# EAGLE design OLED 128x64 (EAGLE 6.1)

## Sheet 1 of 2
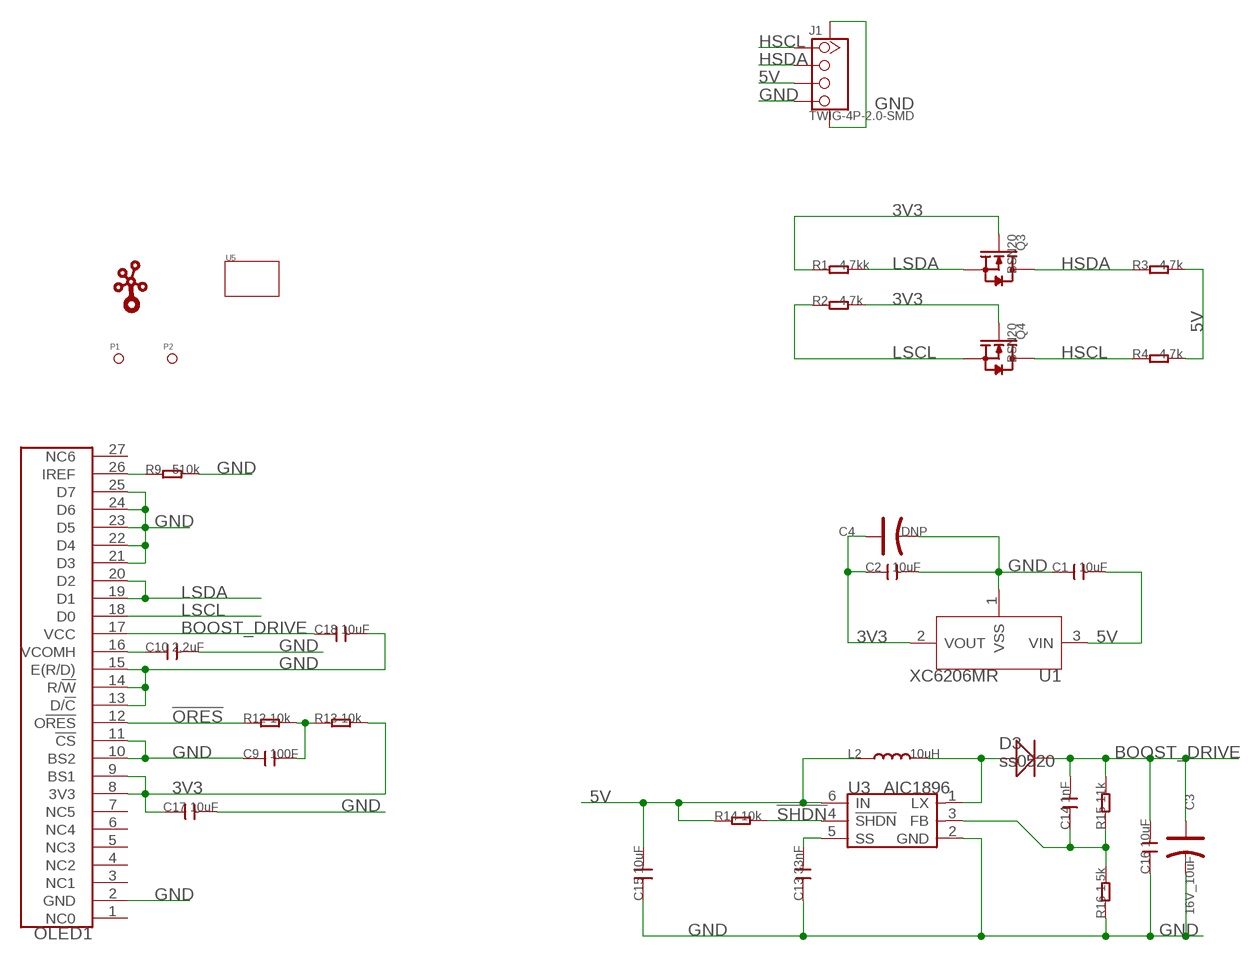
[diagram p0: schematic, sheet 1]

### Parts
C1  10uF  C-0805  [C0805]
C2  10uF  C-0805  [C0805]
C3  16V_10uF  CAP-AVX-A  [AVX-A]
C4  DNP  CAP-AVX-A  [AVX-A]
C9  100F  C-0603  [C0603]
C10  2.2uF  C-0805  [C0805]
C13  33nF  C-0603  [C0603]
C14  1nF  C-0603  [C0603]
C15  10uF  006-C0805  [0805]
C16  10uF  C-0805  [C0805]
C17  10uF  C-0805  [C0805]
C18  10uF  C-0805  [C0805]
D3  ss0520  010-DSOD123  [SOD123]
J1  TWIG-4P-2.0-SMD  TWIG-4P-2.0-SMD-FEMALE-REINFORCE'90D'  [4P-SMD-2.0-90D]
L2  10uH  L'1813'  [1813]
OLED1  OLED_12864BEND  [0LED128X64_BEND]
P1  PAD-MARK  [ROUND-MARK-1.0]
P2  PAD-MARK  [ROUND-MARK-1.0]
Q3  BSN20  MOSFET-N'SOT23'  [SOT23]
Q4  BSN20  MOSFET-N'SOT23'  [SOT23]
R1  4.7kk  R-0603  [R0603]
R2  4.7k  R-0603  [R0603]
R3  4.7k  R-0603  [R0603]
R4  4.7k  R-0603  [R0603]
R9  510k  R-0603  [R0603]
R12  10k  R-0603  [R0603]
R13  10k  R-0603  [R0603]
R14  10k  R-0603  [R0603]
R15  11k  R-0603  [R0603]
R16  1.5k  R-0603  [R0603]
U1  XC6206MR  [SOT23]
U3  AIC1896  [SOT23-6]
U5  TWIG'2U'  [2U-DIM-W/DRILL]
U$1  TWIGLOGOTWIGLOGO_SMALL  [TWIGLOGO_SMALL]

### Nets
3V3: C2.1 C4.+ C17.1 OLED1.8(3V3) OLED1.9(BS1) Q3.1(G) Q4.1(G) R1.1 R2.2 R13.2 U1.2(VOUT)
5V: C1.2 C15.2 J1.3 L2.1 R3.2 R4.2 R14.1 U1.3(VIN) U3.6(IN)
!ORES: OLED1.12(O!RES) R12.1
!SHDN: R14.2 U3.4(!SHDN)
BOOST_DRIVE: C3.+ C14.2 C16.2 C18.1 D3.- OLED1.17(VCC) R15.2
GND: C1.1 C2.2 C3.- C4.- C9.1 C10.2 C13.1 C15.1 C16.1 C17.2 C18.2 J1.4 J1.SS1 J1.SS2 OLED1.2(GND) OLED1.10(BS2) OLED1.11(!CS) OLED1.13(D/!C) OLED1.14(R/!W) OLED1.15(E(R/D)) OLED1.21(D3) OLED1.22(D4) OLED1.23(D5) OLED1.24(D6) OLED1.25(D7) R9.2 R16.1 U1.1(VSS) U3.2(GND)
HSCL: J1.1 Q4.3(D) R4.1
HSDA: J1.2 Q3.3(D) R3.1
LSCL: OLED1.18(D0) Q4.2(S) R2.1
LSDA: OLED1.19(D1) OLED1.20(D2) Q3.2(S) R1.2
N$7: C13.2 U3.5(SS)
N$8: D3.+ L2.2 U3.1(LX)
N$9: C14.1 R15.1 R16.2 U3.3(FB)
N$10: OLED1.26(IREF) R9.1
N$11: C10.1 OLED1.16(VCOMH)
N$12: C9.2 R12.2 R13.1
Unconnected: OLED1.1(NC0) OLED1.3(NC1) OLED1.4(NC2) OLED1.5(NC3) OLED1.6(NC4) OLED1.7(NC5) OLED1.27(NC6)

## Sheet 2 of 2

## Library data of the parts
C1 C2 C9 C10 C13 C14 C16-C18 = Discrete:C*: Ceramic Capacitors
C3 C4 = Discrete:CAP*: Electrolytic Capacitors,Tantalum Capacitors and Super Capacitors
C15 = Discrete:006-C*: Ceramic Capacitors
D3 = Discrete:010-D*
J1 = Connector:TWIG-4P-2.0-SMD-FEMALE-REINFORCE
L2 = Discrete:L*
OLED1 = EXT_moudle:OLED_12864
P1 P2 = Discrete:PAD-MARK; PARTNO: DNP
Q3 Q4 = Discrete:MOSFET-N: IRLL014: http://www.vishay.com/docs/91319/sihll014.pdf
R1-R4 R9 R12-R16 = Discrete:R*
U1 = IC:XC6206: LOW ESR Cap.Compatible Positive Voltage Regulators
U3 = ICs_v54:AIC1896
U5 = moudle:TWIG
U$1 = seeedleo:TWIGLOGO

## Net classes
0 default: width 0.203 mm, drill 0.305 mm, clearance 0.203 mm
1 power: width 0.203 mm, drill 0.305 mm, clearance 0.203 mm
2 gnd: width 0.203 mm, drill 0.305 mm, clearance 0.203 mm
3 usbvcc: width 0.203 mm, drill 0.305 mm, clearance 0.203 mm

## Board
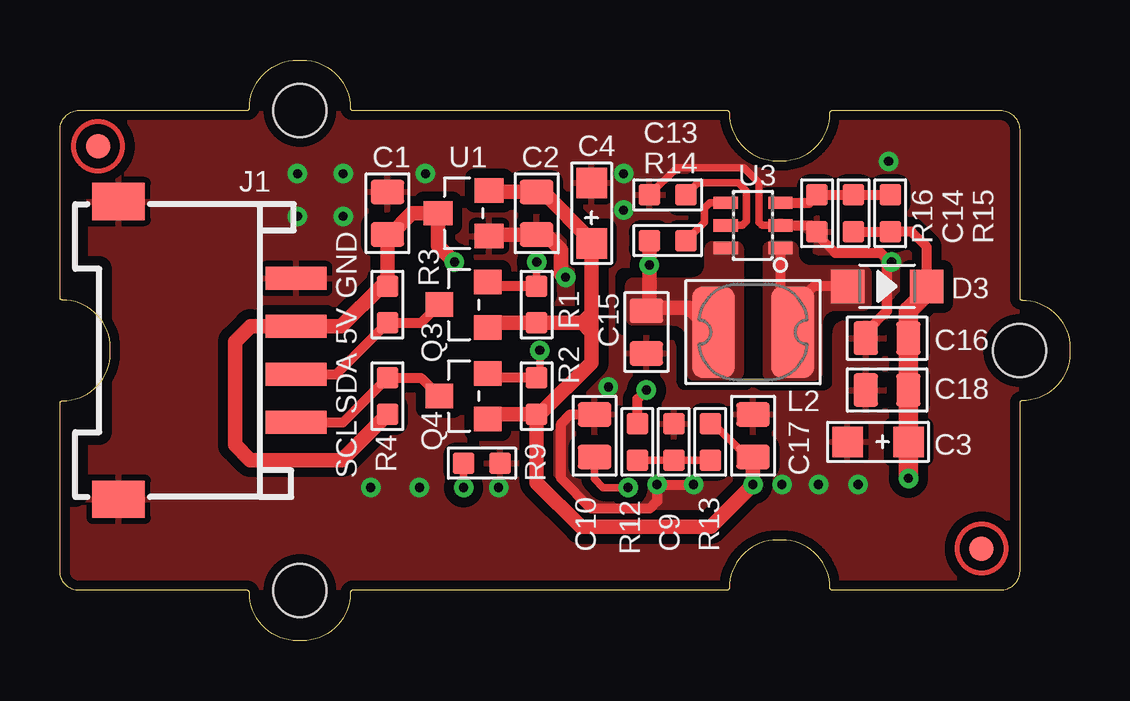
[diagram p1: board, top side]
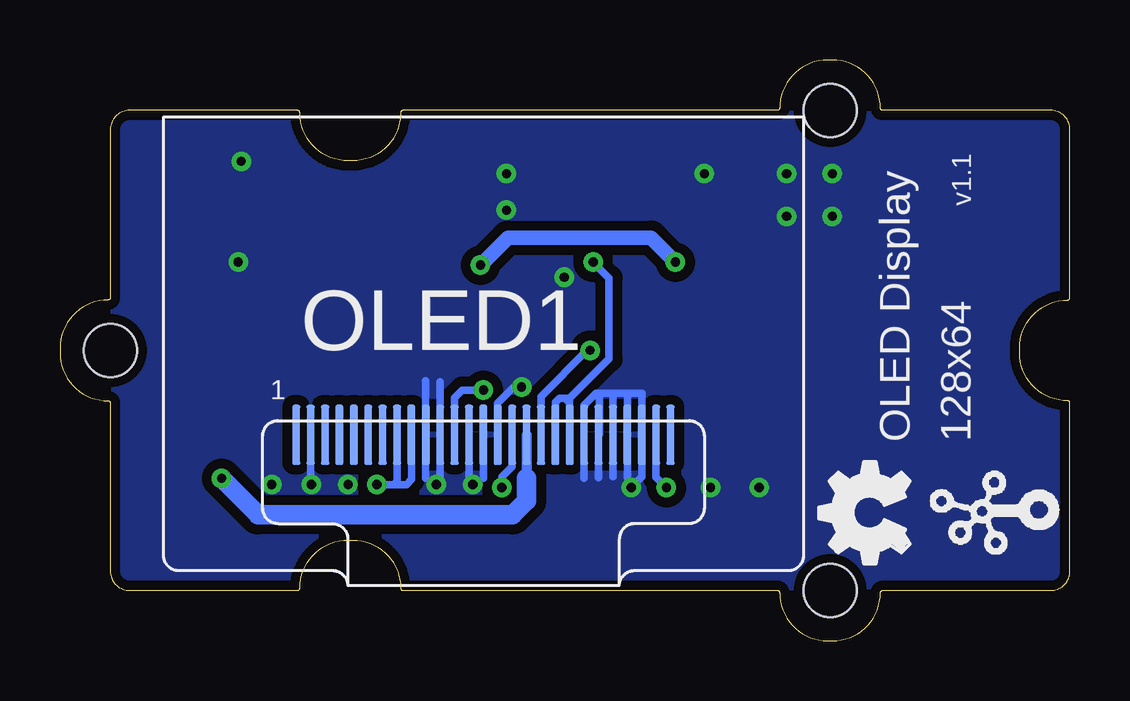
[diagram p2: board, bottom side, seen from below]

Size 42.1 x 24.2 mm. Coordinates in mm from the lower left corner, seen from the top.
Copper layers (1*16): Top 0.035mm / dielectric 1.5mm / Bottom 0.035mm
Design rules: minimum track width 6mil, minimum drill 12mil, track to track 6mil, track to pad 6mil, pad to pad 6mil, via to via 6mil, smd to smd 0mil, copper to edge 10mil, drill to drill 10mil, minimum pad ring 10mil, minimum via ring 6mil, stop-mask expansion 2mil, vias tented up to drill 100mil, thermal gap 10mil
bRestrict: area 24.7,7.9 to 24.8,8.3; area 27.1,7.9 to 27.2,8.3; area 25.3,7.9 to 25.5,8.3; area 18.7,7.9 to 18.9,8.3; area 20.5,7.9 to 20.6,8.3; area 19.9,7.9 to 20,8.3; area 19.4,7.9 to 19.5,8.3; area 38.5,-10.9 to 38.9,-10.6; area 29.5,-15 to 29.9,-14.4; area 27.1,-15 to 28.1,-14.4; area 21,-15 to 23.3,-14.4; area 16.3,-11 to 16.7,-10.5

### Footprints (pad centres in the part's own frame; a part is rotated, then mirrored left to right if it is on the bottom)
C0805 = smd 1.016 x 1.397: 1 -0.889,0; 2 0.889,0
AVX-A = smd 1.27 x 1.27: + -1.27,0; - 1.27,0
C0603 = smd 0.889 x 0.889: 1 -0.762,0; 2 0.762,0
0805 = smd 1.016 x 1.397: 1 -0.889,0; 2 0.889,0
SOD123 = smd 1.397 x 1.397: + 1.651,0; - -1.651,0
4P-SMD-2.0-90D = smd 0.965 x 2.54: 1 -3,0; 2 -1,0; 3 1,0; 4 3,0 | smd 1.55 x 2.184: SS1 -6.2,7.4; SS2 6.2,7.4
1813 = smd 1.778 x 3.81: 1 -1.651,0; 2 1.651,0
0LED128X64_BEND = smd 0.35 x 2.5: 1 -7.805,5.624; 2 -7.205,5.624; 3 -6.605,5.624; 4 -6.005,5.624; 5 -5.405,5.624; 6 -4.805,5.624; 7 -4.205,5.624; 8 -3.605,5.624; 9 -3.005,5.624; 10 -2.405,5.624; 11 -1.805,5.624; 12 -1.205,5.624; 13 -0.605,5.624; 14 -0.005,5.624; 15 0.595,5.624; 16 1.195,5.624; 17 1.795,5.624; 18 2.395,5.624; 19 2.995,5.624; 20 3.595,5.624; 21 4.195,5.624; 22 4.795,5.624; 23 5.395,5.624; 24 5.995,5.624; 25 6.595,5.624; 26 7.195,5.624; 27 7.795,5.624
ROUND-MARK-1.0 = smd 1.016 x 1.016: P$1 0,0
SOT23 = smd 1.016 x 1.143: 1 -0.95,-1.016; 2 0.95,-1.016; 3 0,1.016
R0603 = smd 0.889 x 0.889: 1 -0.762,0; 2 0.762,0
SOT23' = smd 1.016 x 1.2: 1 -0.95,-1.06; 2 0.95,-1.06; 3 0,1.06
SOT23-6 = smd 0.508 x 1.016: 1 -0.94,-1.143; 2 0,-1.143; 3 0.94,-1.143; 4 0.94,1.143; 5 0,1.143; 6 -0.94,1.143
2U-DIM-W/DRILL = hole 2.2: -10,-10; -10,10; 20,0

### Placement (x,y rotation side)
C1  13.65,17.81 270 top
C2  19.87,17.81 270 top
C3  34.1,8.29 180 top
C4  22.16,17.81 90 top
C9  25.59,8.29 270 top
C10  22.29,8.54 90 top
C13  25.33,18.58 0 top
C14  33.08,17.81 270 top
C15  24.45,12.86 90 top
C16  34.48,12.61 0 top
C17  28.89,8.54 90 top
C18  34.48,10.45 180 top
D3  34.48,14.77 180 top
J1  9.84,12.1 90 top
L2  28.89,12.86 0 top
OLED1  24.45,2.96 0 bottom
P1  38.42,3.84 0 top
P2  1.59,20.61 0 top
Q3  16.83,14 90 top
Q4  16.83,10.2 90 top
R1  19.87,14 90 top
R2  19.87,10.2 270 top
R3  13.65,14 90 top
R4  13.65,10.2 270 top
R9  17.59,7.4 0 top
R12  24.06,8.29 270 top
R13  27.11,8.29 90 top
R14  25.33,16.67 0 top
R15  34.61,17.81 270 top
R16  31.56,17.81 90 top
U1  XC6206MR  [SOT23']  16.83,17.81 90 top
U3  28.89,17.31 90 top
U5  20,12.1 180 bottom
U$1  0.32,3.21 90 bottom
U$2  [OSHW_FILLX150_NOTEXT]  6.67,3.21 90 bottom

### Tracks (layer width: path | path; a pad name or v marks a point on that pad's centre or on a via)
3V3  (via drill 0.38 pad 0.81)
  Top 0.305: R13.2 27.24,9.05 28.38,7.91 28.64,7.91 C17.1
  Top 0.61: R2.2 19.87,6.59 21.71,4.75 27.13,4.75 v28.89,6.51 C17.1 | 22.16,12.86 22.16,11.6 20,9.43 R2.2 | U1.2 17.95,18.7 C2.1 20.13,18.7 22.16,16.67 C4.+ 22.16,13.62 | 22.16,13.62 22.16,13.24 | 22.16,13.24 22.16,12.86 | Q3.1 18.03,13.24 R1.1 22.16,13.24 | 22.16,13.62 21.78,13.24 22.16,12.86 | R2.2 18.13,9.43 arc45 17.96,9.36 Q4.1
  Bottom 0.305: OLED1.9 27.45,6.72 27.66,6.51 27.94,6.51 | 27.94,6.51 28,6.51 | 28,6.51 28.19,6.51 | 28.19,6.51 v28.89,6.51 | OLED1.8 28.05,6.65 | 28.05,6.62 28.05,6.56 28,6.51 | 28.05,6.65 28.19,6.51 | 28.05,6.65 28.05,6.62 | 28.05,6.62 27.94,6.51
5V  (via drill 0.38 pad 0.81)
  Top 0.61: 13.65,16.8 C1.2 | R14.1 v24.57,15.66 24.57,13.88 | 24.57,13.88 C15.2 | 24.57,13.88 26.22,13.88 L2.1 | R4.2 11.75,7.53 7.94,7.53 7.3,8.16 7.3,12.47 7.95,13.12 9.82,13.12 J1.3 11.73,13.1 13.4,14.77 R3.2 C1.2 | v16.44,15.78 15.77,16.46 U1.3 14.67,17.81 13.78,16.93 C1.2
  Bottom 0.61: v24.57,15.66 23.43,16.8 17.46,16.8 v16.44,15.78
  pour Top (isolate 0.254, no thermals): 27.24,16.55 28.13,16.55 arc-90 28.38,16.29 28.38,11.21 arc-90 28.13,10.96 26.48,10.96 arc-90 26.22,11.21 26.22,12.61 arc90 25.59,13.24 23.94,13.24 arc-90 23.68,13.5 23.68,14.77 arc-90 23.94,15.02 26.35,15.02 arc90 26.98,15.66 26.98,16.29 arc-90
!ORES  (via drill 0.38 pad 0.81)
  Top 0.406: R12.1 24.06,10.07 v24.45,10.45
  Bottom 0.305: v24.45,10.45 25.33,10.45 25.65,10.13 OLED1.12
!SHDN
  Top 0.305: U3.4 27.09,18.25 26.86,18.01 26.86,17.43 R14.2
BOOST_DRIVE  (via drill 0.38 pad 0.81)
  Top 0.406: C14.2 R15.2 35.49,17.05 36.13,16.42 D3.-
  Top 0.813: D3.- 36.13,14.51 35.37,13.75 C16.2 C18.1 C3.+ v35.37,6.77
  Bottom 0.406: OLED1.17 22.65,6.76 22.65,6.46
  Bottom 0.813: 22.65,6.76 22.65,5.82 23.23,5.24 33.84,5.24 v35.37,6.77
GND  (via drill 0.38 pad 0.81)
  Top 0.305: U3.2 29.27,17.31 29.14,17.43 29.14,19.09 28.51,19.72 25.72,19.72 C13.1
  Top 0.406: U3.2 31.3,17.31 R16.1 31.56,16.93 32.32,16.16 34.22,16.16 34.48,15.91 34.48,13.75 33.59,12.86 C16.1 | C10.2 21.27,9.43 20.89,9.05 20.89,6.77 22.15,5.51 24.59,5.51 24.89,5.81 v24.89,6.51 v26.41,6.51
  Top 0.61: v21.08,15.15 21.02,15.15 20.89,15.27 20.89,16.29 20.25,16.93 C2.2 17.84,16.93
  Bottom 0.305: OLED1.15 23.85,9.9 23.18,10.58 v22.86,10.58 | OLED1.14 24.45,6.77 | 26.86,6.77 OLED1.10 26.86,10.83 | 26.25,6.87 OLED1.11 26.25,10.8 | OLED1.13 25.05,6.8 | 20.25,6.77 OLED1.21 20.25,9.81 19.75,10.32 19.62,10.32 | 18.45,6.79 OLED1.24 18.45,10.3 18.48,10.32 | 19.05,6.83 OLED1.23 19.05,10.26 18.98,10.32 | 19.65,6.8 OLED1.22 19.62,8.61 19.62,10.32 | OLED1.2 31.65,6.55 31.68,6.51 | 17.95,6.72 v18.29,6.38 17.84,6.83 OLED1.25 17.84,10.32 18.48,10.32 | 18.48,10.32 18.98,10.32 | 18.98,10.32 19.62,10.32
  other vias: 23.49,17.94 23.49,19.47 15.24,19.47 11.81,19.47 11.81,17.69 30.1,6.51 31.62,6.51 33.27,6.51 14.98,6.38 12.95,6.38 34.67,15.78 34.54,19.97 9.9,19.47 9.9,17.69
  pour Top: -4.13,20.23 -5.65,20.23 -5.65,18.58 -4.13,18.58
  pour Top (isolate 0.406, rank 6): 42.23,24.29 -0.95,24.29 -0.95,0.04 42.23,0.04
  pour Bottom (isolate 0.406): 42.23,24.29 -0.95,24.29 -0.95,0.04 42.23,0.04
HSCL
  Top 0.406: Q4.3 15.05,10.96 R4.1 11.79,9.1 J1.1
HSDA
  Top 0.406: Q3.3 15.05,13.24 R3.1 11.51,11.1 J1.2
LSCL  (via drill 0.38 pad 0.81)
  Top 0.305: v20,12.1 20,11.08 R2.1
  Top 0.406: R2.1 18.03,10.96 Q4.2
  Bottom 0.305: OLED1.18 22.05,10.18 20.13,12.1 v20,12.1
LSDA  (via drill 0.38 pad 0.81)
  Top 0.305: v19.87,15.78 R1.2
  Top 0.406: R1.2 18.03,14.77 Q3.2
  Bottom 0.305: OLED1.20 20.85,10.11 | 20.85,10.11 19.21,11.75 19.21,15.12 v19.87,15.78 | 20.85,10.11 21.01,10.11 | 21.01,10.11 21.28,10.11 21.45,9.93 OLED1.19 | 21.01,10.11 21.01,10.06 20.89,9.94
N$7
  Top 0.305: U3.5 28.45,17.31 28.62,17.48 28.62,18.74 28.27,19.09 26.6,19.09 C13.2
N$8
  Top 0.406: U3.1 30.03,14.13 | 30.03,14.13 30.03,13.37 L2.2 | D3.+ 31.43,14.77 30.8,14.13 30.03,14.13
  pour Top (isolate 0.254, no thermals): 30.67,16.16 30.67,16.29 arc90 30.41,16.55 29.65,16.55 arc90 29.4,16.29 29.4,11.21 arc90 29.65,10.96 31.43,10.96 arc90 31.68,11.21 31.68,13.24 arc-90 32.32,13.88 33.46,13.88 arc90 33.72,14.13 33.72,15.27 arc90 33.46,15.53 31.3,15.53 arc-90
N$9
  Top 0.406: U3.3 31.23,18.25 R16.2 C14.1 R15.1
N$10  (via drill 0.38 pad 0.81)
  Top 0.305: v16.83,6.38 R9.1
  Bottom 0.305: OLED1.26 17.25,6.81 v16.83,6.38
N$11  (via drill 0.38 pad 0.81)
  Top 0.305: C10.1 22.29,6.74 22.65,6.38 v23.68,6.38
  Bottom 0.305: OLED1.16 23.25,7.26 23.68,6.83 v23.68,6.38
N$12
  Top 0.305: R12.2 C9.2 R13.1

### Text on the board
tPlace: GND | 5V | SDA | SCL
bPlace: v1.1 | 128x64 | OLED Display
